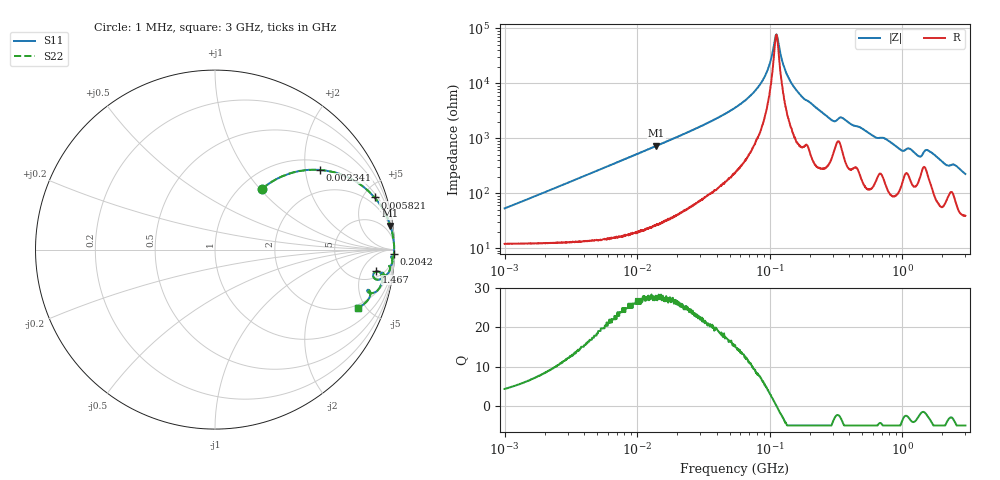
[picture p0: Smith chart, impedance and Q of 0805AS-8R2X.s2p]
!s-Parameter Generated by FASTRON Sdn. Bhd.
!FASTRON P/N : 0805AS-8R2X
!Keysight Technologies: E4991B_MY54100416_A.01.15
!Date: Mon Jun 15 13:00:00 2026
!Version  :Rev01  Mon Jun 15 13:00:00 2026
!Data & Calibration Information:
!Freq  S11  S21  S12  S22
!PortZ  Port1:50+j0  Port2:50+j0
!When reading reference impedance value at option line is always used.
! Remarks : This data is being provided solely for informational purposes.
# Hz S dB R 50
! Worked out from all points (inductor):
!   1601 points, 1 MHz to 3 GHz, reference 50 ohm
!   read as one part in series: L = 8.2 uH near 1.041 MHz
!   highest Q = 27.7 at 13.97 MHz (marker M1), where L = 8.32 uH
!   self-resonance near 112 MHz
!   S11 on the Smith chart (normalised r, x): 1 MHz: 1.24, +1.03; 2.341 MHz: 1.25, +2.41; 5.821 MHz: 1.30, +6.01; 204.2 MHz: 11, -87; 1.467 GHz: 7, -10; 3 GHz: 1.78, -4.41
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1000000  -7.34 52.2  -1.82 -24.7  -1.82 -24.7  -7.34 52.2
2341230  -2.67 37.1  -4.34 -47.0  -4.34 -47.0  -2.67 37.1
3804036  -1.23 26.2  -7.09 -60.0  -7.09 -60.0  -1.23 26.2
5820586  -0.58 18.1  -10.10 -69.1  -10.10 -69.1  -0.58 18.1
1.397259e7  -0.12 7.8  -17.40 -80.1  -17.40 -80.1  -0.12 7.8
1.447069e7  -0.12 7.5  -17.70 -80.4  -17.70 -80.4  -0.12 7.5
5.504702e7  -0.02 1.6  -31.20 -84.7  -31.20 -84.7  -0.02 1.6
8.810787e7  -0.01 0.5  -40.90 -80.4  -40.90 -80.4  -0.01 0.5
9.885493e7  -0.01 0.3  -46.40 -73.9  -46.40 -73.9  -0.01 0.3
1.092603e8  -0.01 0.1  -55.70 -39.0  -55.70 -39.0  -0.01 0.1
1.125904e8  -0.01 -0.0  -57.80 1.5  -57.80 1.5  -0.01 -0.0
1.282345e8  -0.01 -0.3  -46.00 74.1  -46.00 74.1  -0.01 -0.3
1.410248e8  -0.01 -0.5  -41.40 79.9  -41.40 79.9  -0.01 -0.5
1.714156e8  -0.02 -0.9  -35.70 82.4  -35.70 82.4  -0.02 -0.9
2.042267e8  -0.02 -1.3  -32.80 82.2  -32.80 82.2  -0.02 -1.3
2.083556e8  -0.02 -1.4  -32.50 82.8  -32.50 82.8  -0.02 -1.4
2.987278e8  -0.10 -2.6  -26.50 74.0  -26.50 74.0  -0.10 -2.6
3.523638e8  -0.10 -2.3  -27.50 73.1  -27.50 73.1  -0.10 -2.3
7.925923e8  -0.16 -6.3  -19.20 77.1  -19.20 77.1  -0.16 -6.3
1.327057e9  -0.74 -10.5  -14.30 59.8  -14.30 59.8  -0.74 -10.5
1.466741e9  -0.84 -7.7  -16.00 50.5  -16.00 50.5  -0.84 -7.7
3e9  -1.32 -22.2  -8.32 57.8  -8.32 57.8  -1.32 -22.2
